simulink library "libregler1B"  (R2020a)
settings: Solver=ode45  StartTime=0.0  StopTime=10.0  RelTol=1e-3

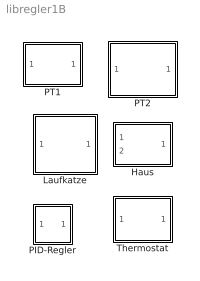
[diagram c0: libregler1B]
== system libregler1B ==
  Haus : Subsystem  mask(Regelstrecke Haus){C=100000, R=0.001, T0=16}
      mask prompts: C "Waermekapazitaet"; R "Waermewiderstand"; T0 "Anfangstemperatur"
      mask help: Temperatur eines Hauses als Regelstrecke. Aussentemperatur als Stoergroesse
  Laufkatze : Subsystem  mask(Laufkatze){mk=100, ml=10, l=1}
      mask prompts: mk "Laufkatzenmasse mk"; ml "Lastmasse ml"; l "Seillaenge l"
      mask help: Modell einer Laufkatze als Regelstrecke
  PID-Regler : Subsystem  mask(PID-Regler){Kp=1, Ki=1, Kd=0}
      mask prompts: Kp "Proportional:"; Ki "Integral:"; Kd "Ableitung:"
      mask help: Regler mit Proportional-, Integral- und Ableitungsanteil.
  PT1 : Subsystem  mask(PT1){T=2, Kp=5}
      mask prompts: T "Verzoegerungszeit T"; Kp "Verstaerkung Kp"
      mask help: Regelstrecke: einfaches Verzoegerungsglied vom PT1-Typ
  PT2 : Subsystem  mask(PT2){D=0.2, om0=1.0, b0=1.0}
      mask prompts: D "Daempfungsgrad"; om0 "Eigenfrequenz"; b0 "Staerke"
      mask help: schwingfaehige Regelstrecke mit Daempfung D Eigenfrequenz om0 Starke b0
  Thermostat : Subsystem  mask{umax=18500, delta=0.5}
      mask prompts: umax "Schaltwert"; delta "Ausschalt-Hysterese"

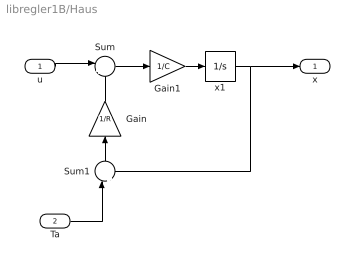
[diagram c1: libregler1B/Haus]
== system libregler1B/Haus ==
  u : Inport
  Ta : Inport  Port=2
  Gain : Gain  Gain=1/R  SaturateOnIntegerOverflow=on
  Gain1 : Gain  Gain=1/C  SaturateOnIntegerOverflow=on
  Sum : Sum  Inputs=|++  SaturateOnIntegerOverflow=on
  Sum1 : Sum  Inputs=|+-  SaturateOnIntegerOverflow=on
  x1 : Integrator  InitialCondition=T0
  x : Outport
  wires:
  Gain1/1 -> x1/1
  Sum/1 -> Gain1/1
  x1/1 -> x/1, Sum1/2
  u/1 -> Sum/1
  Gain/1 -> Sum/2
  Sum1/1 -> Gain/1
  Ta/1 -> Sum1/1

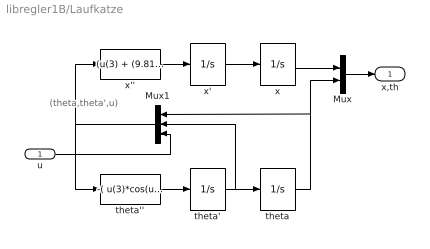
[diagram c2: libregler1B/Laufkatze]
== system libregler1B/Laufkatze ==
  note: (theta,theta',u)
  u : Inport
  Mux : Mux  Inputs=2
  Mux1 : Mux  Inputs=3
  theta : Integrator
  theta' : Integrator
  theta'' : Fcn  Expr=-( u(3)*cos(u(1)) + (9.81+ l*u(2)^2*cos(u(1)))*ml*sin(u(1)) + 9.81*mk*sin(u(1)) ) / ( (mk + ml*sin(u(1))^2)*l )
  x : Integrator
  x' : Integrator
  x'' : Fcn  Expr=(u(3) + (9.81*cos(u(1)) + l*u(2)^2)*ml*sin(u(1)))/(mk + ml*sin(u(1))^2)
  x,th : Outport
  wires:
  Mux/1 -> x,th/1
  x/1 -> Mux/1
  theta/1 -> Mux/2, Mux1/1
  Mux1/1 -> x''/1, theta''/1
  x'/1 -> x/1
  theta'/1 -> theta/1, Mux1/2
  u/1 -> Mux1/3
  x''/1 -> x'/1
  theta''/1 -> theta'/1

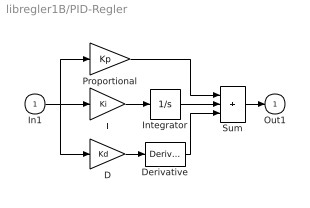
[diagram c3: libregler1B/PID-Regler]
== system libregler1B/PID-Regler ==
  In1 : Inport
  D : Gain  Gain=Kd  SaturateOnIntegerOverflow=on
  Derivative : Derivative
  I : Gain  Gain=Ki  SaturateOnIntegerOverflow=on
  Integrator : Integrator
  Proportional : Gain  Gain=Kp  SaturateOnIntegerOverflow=on
  Sum : Sum  Inputs=+++  InputSameDT=on  SaturateOnIntegerOverflow=on
  Out1 : Outport  InitialOutput=0
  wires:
  D/1 -> Derivative/1
  Sum/1 -> Out1/1
  In1/1 -> D/1, Proportional/1, I/1
  Derivative/1 -> Sum/3
  Integrator/1 -> Sum/2
  Proportional/1 -> Sum/1
  I/1 -> Integrator/1

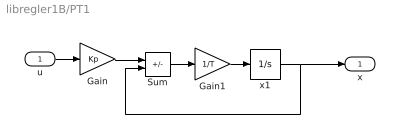
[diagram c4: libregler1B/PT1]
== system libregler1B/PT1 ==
  u : Inport
  Gain : Gain  Gain=Kp  SaturateOnIntegerOverflow=on
  Gain1 : Gain  Gain=1/T  SaturateOnIntegerOverflow=on
  Sum : Sum  Inputs=+-  SaturateOnIntegerOverflow=on
  x1 : Integrator
  x : Outport
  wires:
  u/1 -> Gain/1
  Gain/1 -> Sum/1
  x1/1 -> x/1, Sum/2
  Sum/1 -> Gain1/1
  Gain1/1 -> x1/1

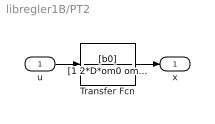
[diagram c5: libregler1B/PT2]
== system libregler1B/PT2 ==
  u : Inport
  Transfer Fcn : TransferFcn  Numerator=[b0]  Denominator=[1 2*D*om0 om0*om0]
  x : Outport
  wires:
  u/1 -> Transfer Fcn/1
  Transfer Fcn/1 -> x/1

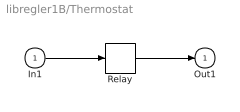
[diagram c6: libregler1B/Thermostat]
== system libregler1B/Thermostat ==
  In1 : Inport
  Relay : Relay  OnSwitchValue=0  OffSwitchValue=-delta  OnOutputValue=umax
  Out1 : Outport  InitialOutput=0
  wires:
  In1/1 -> Relay/1
  Relay/1 -> Out1/1
